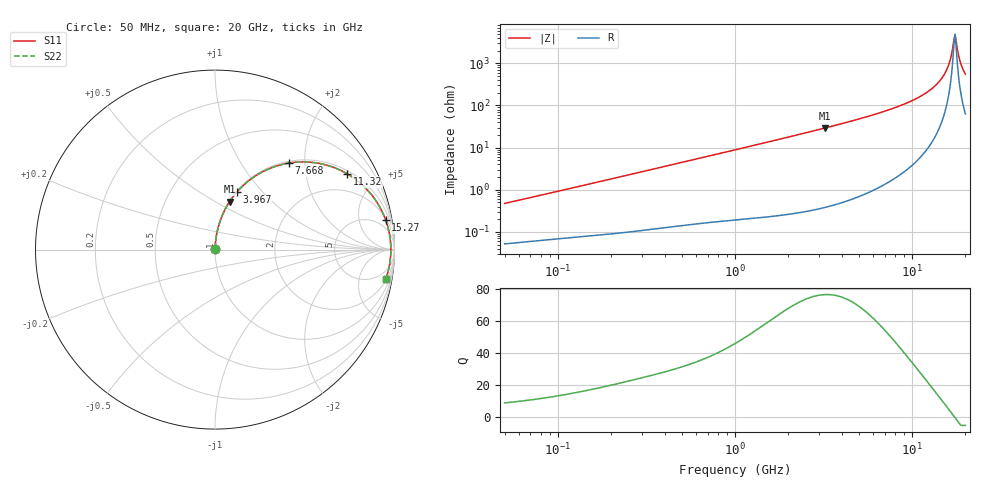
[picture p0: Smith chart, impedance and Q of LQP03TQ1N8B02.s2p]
!Murata Part Number: LQP03TQ1N8B02
!These Parameters are Measured in Series Mode Connection
!  o--[Z]--o
!Port1  Port2
!  o-------o
!Freq. Start=50[MHz] Stop=20[GHz], 401[Steps]
# Hz S RI R 50
!Freq.(Hz) S11(Real) S11(Imag) S21(Real) S21(Imag) S12(Real) S12(Imag) S22(Real) S22(Imag)
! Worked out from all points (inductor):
!   401 points, 50 MHz to 20 GHz, reference 50 ohm
!   read as one part in series: L = 1.48 nH near 51.52 MHz
!   highest Q = 76.7 at 3.217 GHz (marker M1), where L = 1.44 nH
!   self-resonance near 17.22 GHz
!   S11 on the Smith chart (normalised r, x): 50 MHz: 1.00, +0.01; 3.967 GHz: 1.01, +0.73; 7.668 GHz: 1.03, +1.66; 11.32 GHz: 1.13, +3.41; 15.27 GHz: 2, +11; 20 GHz: 2, -11
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5e7  0.00054 0.0047  0.9995 -0.0047  0.9995 -0.0047  0.00054 0.0047
1.364002e8  0.000918 0.0124  0.9991 -0.0124  0.9991 -0.0124  0.000918 0.0124
3.721004e8  0.00231 0.0331  0.9977 -0.0331  0.9977 -0.0331  0.00231 0.0331
1e9  0.0096 0.0873  0.9904 -0.0873  0.9904 -0.0873  0.0096 0.0873
2.728004e9  0.0593 0.2296  0.9407 -0.2296  0.9407 -0.2296  0.0593 0.2296
3.216634e9  0.0812 0.2668  0.9188 -0.2668  0.9188 -0.2668  0.0812 0.2668
3.967106e9  0.1214 0.3201  0.8786 -0.3201  0.8786 -0.3201  0.1214 0.3201
5.515528e9  0.2267 0.4112  0.7733 -0.4112  0.7733 -0.4112  0.2267 0.4112
7.442007e9  0.3897 0.478  0.6103 -0.478  0.6103 -0.478  0.3897 0.478
7.668323e9  0.4104 0.4819  0.5896 -0.4819  0.5896 -0.4819  0.4104 0.4819
9.457416e9  0.5762 0.4811  0.4238 -0.4811  0.4238 -0.4811  0.5762 0.4811
1.131968e10  0.7369 0.4221  0.2631 -0.4221  0.2631 -0.4221  0.7369 0.4221
1.354865e10  0.8839 0.2904  0.1161 -0.2904  0.1161 -0.2904  0.8839 0.2904
1.527346e10  0.9514 0.1636  0.0486 -0.1636  0.0486 -0.1636  0.9514 0.1636
1.597544e10  0.9671 0.1102  0.0329 -0.1102  0.0329 -0.1102  0.9671 0.1102
1.646126e10  0.9742 0.0734  0.0258 -0.0734  0.0258 -0.0734  0.9742 0.0734
1.696185e10  0.9784 0.0361  0.0216 -0.0361  0.0216 -0.0361  0.9784 0.0361
1.747767e10  0.9798 -0.0015  0.0202 0.0015  0.0202 0.0015  0.9798 -0.0015
1.800918e10  0.9783 -0.0391  0.0217 0.0391  0.0217 0.0391  0.9783 -0.0391
1.88369e10  0.9706 -0.0949  0.0294 0.0949  0.0294 0.0949  0.9706 -0.0949
1.940974e10  0.9621 -0.1312  0.0379 0.1312  0.0379 0.1312  0.9621 -0.1312
2e10  0.9508 -0.1665  0.0492 0.1665  0.0492 0.1665  0.9508 -0.1665
